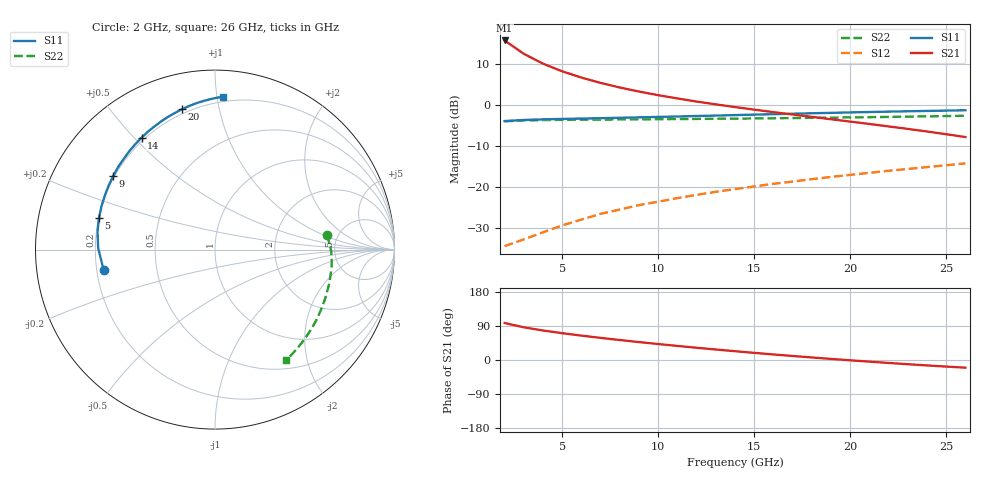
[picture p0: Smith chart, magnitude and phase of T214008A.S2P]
!AT-21400
!S-PARAMETERS at Vce=8V  Ic=14mA.  LAST UPDATED 07-21-92
# ghz s ma r 50
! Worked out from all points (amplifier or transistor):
!   25 points, 2 GHz to 26 GHz, reference 50 ohm
!   highest |S21| = 15.6 dB at 2 GHz (marker M1)
!   |S21| within 3 dB of that: start of sweep to 2.922 GHz
!   unconditionally stable (mu >= 1): start of sweep to 12.69 GHz
!   at 6 GHz: K = 1.44, MAG = 13.3 dB, |S12| = -28.0 dB
!   at 14 GHz: K = 0.91, MSG = 10.0 dB, |S12| = -20.5 dB
!   at 26 GHz: K = 0.26, MSG = 3.2 dB, |S12| = -14.3 dB
!   S11 on the Smith chart (normalised r, x): 2 GHz: 0.23, -0.08; 5 GHz: 0.20, +0.13; 9 GHz: 0.19, +0.31; 14 GHz: 0.19, +0.53; 20 GHz: 0.18, +0.78; 26 GHz: 0.17, +1.04
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2  0.631 -169.8  6.03 97.6  0.019 23.6  0.627 7.7
3  0.651 179.2  4.146 86.3  0.023 41.9  0.643 2.0
4  0.662 171.4  3.151 77.9  0.028 52.5  0.649 -2.0
5  0.67 164.9  2.541 70.8  0.034 59.1  0.653 -5.2
6  0.677 159.1  2.132 64.4  0.04 63.4  0.656 -8.1
7  0.684 153.8  1.837 58.4  0.047 66.4  0.658 -10.7
8  0.692 148.8  1.615 52.7  0.053 68.5  0.66 -13.2
9  0.7 144.1  1.442 47.3  0.06 70.1  0.663 -15.7
10  0.709 139.6  1.303 42.1  0.066 71.2  0.665 -18.0
11  0.717 135.2  1.188 37.1  0.073 72.1  0.667 -20.4
12  0.727 131.1  1.09 32.3  0.08 72.7  0.67 -22.7
13  0.736 127.1  1.007 27.7  0.087 73.1  0.673 -25.1
14  0.746 123.3  0.934 23.2  0.094 73.4  0.676 -27.4
15  0.756 119.6  0.869 18.9  0.101 73.5  0.679 -29.7
16  0.765 116.1  0.811 14.7  0.109 73.6  0.683 -32.1
17  0.775 112.6  0.758 10.6  0.116 73.5  0.687 -34.5
18  0.785 109.4  0.71 6.7  0.124 73.4  0.691 -36.9
19  0.794 106.2  0.664 2.9  0.132 73.2  0.695 -39.3
20  0.804 103.1  0.622 -0.8  0.14 72.9  0.699 -41.8
22  0.822 97.3  0.543 -7.8  0.157 72.1  0.709 -46.8
24  0.838 91.9  0.471 -14.3  0.174 71.1  0.72 -52.0
26  0.854 86.9  0.403 -20.3  0.193 69.9  0.732 -57.4
